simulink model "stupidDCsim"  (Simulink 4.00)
settings: Solver=ode45  SolverMode=SingleTasking  StartTime=0.0  StopTime=100  RelTol=1e-3  AbsTol=1e-6
PostLoadFcn:
  | stupidDCpostloadfcn
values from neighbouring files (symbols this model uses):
  Ts = 0.01    [pidDCpostloadfcn.m]    (also in stupidDCpostloadfcn.m = 0.1)
undefined symbols (not defined in the file or in its folder): conv, polyc2d, polyval
libraries: adaptlib x3, simulink3 x1

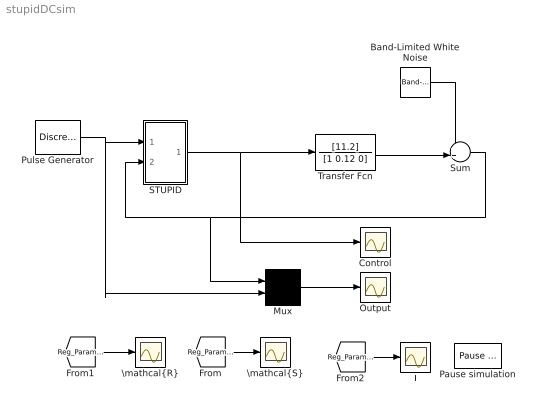
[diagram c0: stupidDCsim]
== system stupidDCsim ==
  Band-Limited White Noise : simulink3/Sources/Band-Limited White Noise  Cov=[0.0001]  Ts=0.1  seed=[23341]
  Control : Scope
  Mux : Mux  Inputs=2
  Output : Scope
  Pause simulation : adaptlib/Pause simulation  par=[50]
  Pulse Generator : DiscretePulseGenerator  PulseType=Time-based  Amplitude=2  Period=10  PulseWidth=50  PhaseDelay=0  SampleTime=1
  STUPID : Subsystem  mask{wo=5, zeta=1, theta0=[0.3;0.1;2; -2], P0=1000*diag([1 1 1 1]), lambda=, a_o=, h=Ts, d0=, um=10}
      mask prompts: wo "w_o (closed loop bandwidth)"; zeta "Closed loop damping"; theta0 "Initial estimate"; P0 "Initial covariance matrix"; lambda "Forgeting factor"; a_o "Observer pole"; h "Sampling time"; d0 "d0 (prediction horizon)"; um "Maximum control signal"
      mask help: DSTR with integral term.
      mask init:
      | Ts=0.1;
  Sum : Sum  Inputs=++|  SaturateOnIntegerOverflow=on
  T : Scope
  Transfer Fcn : TransferFcn  Numerator=[11.2]  Denominator=[1 0.12 0]  AbsoluteTolerance=auto  Realization=auto
  "\\mathcal{R}" : Scope
  "\\mathcal{S}" : Scope
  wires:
  Mux/1 -> Output/1
  Pulse Generator/1 -> Mux/2, STUPID/1(u_c)
  STUPID/1(u) -> Control/1, Transfer Fcn/1
  Transfer Fcn/1 -> Sum/2
  Sum/1 -> STUPID/2(y), Mux/1
  Band-Limited White Noise/1 -> Sum/1
  [Reg_ParametersStilde] -> "\\mathcal{S}"/1
  [Reg_ParametersRtilde] -> "\\mathcal{R}"/1
  [Reg_ParametersT] -> T/1

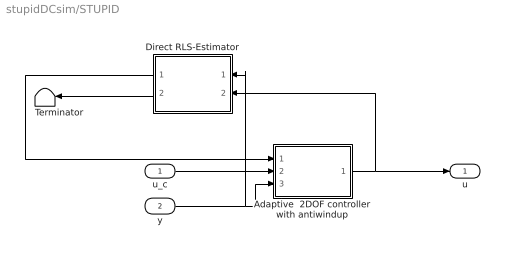
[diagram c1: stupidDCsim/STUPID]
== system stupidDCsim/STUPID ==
  u_c : Inport  Port=1  LatchInput=off
  y : Inport  Port=2  LatchInput=off
  Adaptive  2DOF controller with antiwindup : Subsystem  AncestorBlock=|  mask{n_r=2, ulim=um, A_m=polyc2d([1 2*zeta*wo wo^2],h), A_o=[1 -a_o], A_ow=polyc2d([1 2*0.7*7 7^2],h), h=h}
      | adaptlib/Adaptive 
      | 2DOF controller
      | with antiwindup
      mask prompts: n_r "n_r (degree of R, S and T)"; ulim "Maximum control signal"; A_o "A_o (Observer polynomial)"; A_ow "A_ow (Anti windup polynomial)"; h "Sampling period"
      mask help: A two-degree-of-freedom linear controller with control signal saturation and anti windup. A_o(q)v(k)=T(q)u_c(k)-S(q)y(k)-(A_o(q)-R(q))u(t) u(k)=f(v(k))
  Direct RLS-Estimator : Subsystem  Orientation=left  Priority=1  AncestorBlock=adaptlib/Direct RLS-Estimator  mask{n_r=1, theta_0=theta0, P_0=P0, lambda=lambda, A_m=polyc2d([1 2*zeta*wo wo^2],h), A_o=[1 -a_o], d0=d0, h=h}
      mask prompts: n_r "n_r (degree of estimated R, S )"; theta_0 "Initial estimate"; P_0 "Initial covariance matrix"; h "Sampling period"
  Terminator : Terminator
  u : Outport  Port=1
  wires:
  Direct RLS-Estimator/2(P) -> Terminator/1
  Direct RLS-Estimator/1("[R,S,T]") -> Adaptive  2DOF controller with antiwindup/1("[R,S,T]")
  u_c/1 -> Adaptive  2DOF controller with antiwindup/2(u_c)
  y/1 -> Adaptive  2DOF controller with antiwindup/3(y), Direct RLS-Estimator/1(y)
  Adaptive  2DOF controller with antiwindup/1(u) -> Direct RLS-Estimator/2(u), u/1

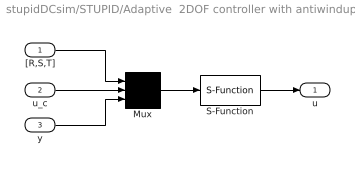
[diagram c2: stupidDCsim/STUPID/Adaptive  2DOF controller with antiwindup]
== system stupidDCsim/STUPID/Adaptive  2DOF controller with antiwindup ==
  "[R,S,T]" : Inport  Port=1  LatchInput=off
  u_c : Inport  Port=2  LatchInput=off
  y : Inport  Port=3  LatchInput=off
  Mux : Mux  Inputs=3
  S-Function : S-Function  FunctionName=rstdirint  Parameters=2,h,A_o,A_ow,A_m,ulim  PortCounts=[]  SFunctionModules=''
  u : Outport  Port=1  InitialOutput=0
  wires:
  "[R,S,T]"/1 -> Mux/1
  y/1 -> Mux/3
  Mux/1 -> S-Function/1
  S-Function/1 -> u/1
  u_c/1 -> Mux/2

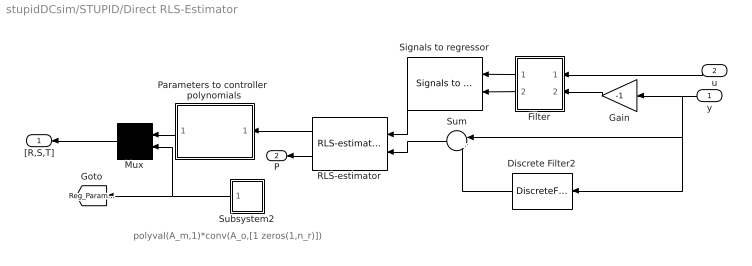
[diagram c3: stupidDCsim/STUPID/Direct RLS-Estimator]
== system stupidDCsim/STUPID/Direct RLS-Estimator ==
  note: polyval(A_m,1)*conv(A_o,[1 zeros(1,n_r)])
  y : Inport  Orientation=left  Port=1  LatchInput=off
  u : Inport  Orientation=left  Port=2  LatchInput=off
  Discrete Filter2 : DiscreteFilter  Orientation=left  Numerator=[zeros(1,d0) 1]*polyval(A_m,1)*polyval(A_o,1)  Denominator=conv(A_m,A_o)  SampleTime=h  Realization=auto
  Filter : Subsystem  Orientation=left  mask{A_m=A_m, A_o=A_o, d0=d0, h=h}
  Gain : Gain  Orientation=left  Gain=-1  Multiplication=Element-wise(K.*u)  SaturateOnIntegerOverflow=on
  Mux : Mux  Orientation=left  Inputs=2
  Parameters to controller  polynomials : Subsystem  Orientation=left  AncestorBlock="adaptlib/Parameters to controller  polynomials"  mask{n_r=n_r}
      mask prompts: n_r "n_r (degree of R, S )"
  RLS-estimator : adaptlib/RLS-estimator  Orientation=left  n=2*(n_r+1)  theta_0=theta_0  P_0=P_0  lambda=lambda  h=h
  Signals to regressor : adaptlib/Signals to regressor  Orientation=left  m=n_r+1  n=n_r+1  h=h
  Subsystem2 : Subsystem  Orientation=left
  Sum : Sum  Orientation=left  Inputs=|+-  SaturateOnIntegerOverflow=on
  "[R,S,T]" : Outport  Orientation=left  Port=1  InitialOutput=0
  P : Outport  Orientation=left  Port=2  InitialOutput=0
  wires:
  Mux/1 -> "[R,S,T]"/1
  Gain/1 -> Filter/2(y)
  u/1 -> Filter/1(u)
  y/1 -> Gain/1, Sum/1, Discrete Filter2/1
  Filter/1(u_f) -> Signals to regressor/1
  Filter/2(y_f) -> Signals to regressor/2
  Signals to regressor/1 -> RLS-estimator/1
  RLS-estimator/2 -> P/1
  RLS-estimator/1 -> Parameters to controller  polynomials/1(theta)
  Parameters to controller  polynomials/1("[R,S]") -> Mux/1
  Sum/1 -> RLS-estimator/2
  Discrete Filter2/1 -> Sum/2
  Subsystem2/1(Out1) -> Mux/2, [Reg_ParametersT]

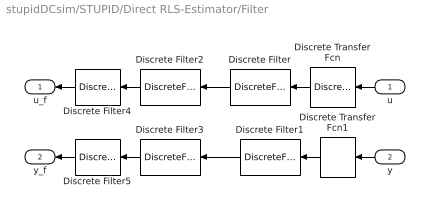
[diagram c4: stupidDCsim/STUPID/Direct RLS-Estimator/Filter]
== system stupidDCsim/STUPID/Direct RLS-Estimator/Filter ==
  u : Inport  Orientation=left  Port=1  LatchInput=off
  y : Inport  Orientation=left  Port=2  LatchInput=off
  Discrete Transfer Fcn : DiscreteTransferFcn  Orientation=left  Numerator=[1]  Denominator=[1 zeros(1,d0) ]  SampleTime=h  Realization=auto
  Discrete Transfer Fcn1 : DiscreteTransferFcn  Orientation=left  Numerator=[1]  Denominator=[1 zeros(1,d0) ]  SampleTime=h  Realization=auto
  Discrete Filter : DiscreteFilter  Orientation=left  Numerator=[1]  Denominator=A_o  SampleTime=h  Realization=auto
  Discrete Filter1 : DiscreteFilter  Orientation=left  Numerator=[1]  Denominator=A_o  SampleTime=h  Realization=auto
  Discrete Filter2 : DiscreteFilter  Orientation=left  Numerator=[1]  Denominator=A_m  SampleTime=h  Realization=auto
  Discrete Filter3 : DiscreteFilter  Orientation=left  Numerator=[1]  Denominator=A_m  SampleTime=h  Realization=auto
  Discrete Filter4 : DiscreteFilter  Orientation=left  Numerator=[1 -1]  Denominator=[1]  SampleTime=h  Realization=auto
  Discrete Filter5 : DiscreteFilter  Orientation=left  Numerator=[1 -1]  Denominator=[1 ]  SampleTime=h  Realization=auto
  u_f : Outport  Orientation=left  Port=1  InitialOutput=0
  y_f : Outport  Orientation=left  Port=2  InitialOutput=0
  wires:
  Discrete Filter2/1 -> Discrete Filter4/1
  Discrete Filter3/1 -> Discrete Filter5/1
  u/1 -> Discrete Transfer Fcn/1
  y/1 -> Discrete Transfer Fcn1/1
  Discrete Filter/1 -> Discrete Filter2/1
  Discrete Filter1/1 -> Discrete Filter3/1
  Discrete Transfer Fcn/1 -> Discrete Filter/1
  Discrete Transfer Fcn1/1 -> Discrete Filter1/1
  Discrete Filter4/1 -> u_f/1
  Discrete Filter5/1 -> y_f/1

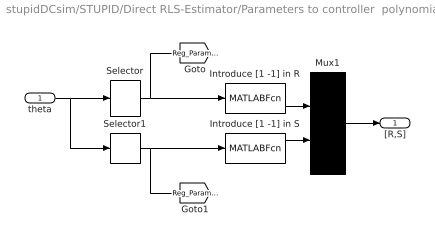
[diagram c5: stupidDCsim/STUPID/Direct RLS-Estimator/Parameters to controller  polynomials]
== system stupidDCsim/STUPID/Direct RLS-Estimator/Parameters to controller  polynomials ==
  theta : Inport  Port=1  LatchInput=off
  Introduce [1 -1] in R : MATLABFcn  MATLABFcn=conv(u,[1 -1])  OutputDimensions=3  OutputSignalType=auto  Output1D=on
  Introduce [1 -1] in S : MATLABFcn  MATLABFcn=conv(u,[1 -1])  OutputDimensions=3  OutputSignalType=auto  Output1D=on
  Mux1 : Mux  Inputs=2
  Selector : Selector  InputType=Vector  ElementSrc=Internal  Elements=[1 : n_r+1]  RowSrc=Internal  Rows=1  ColumnSrc=Internal  Columns=1  InputPortWidth=2*(n_r+1)
  Selector1 : Selector  InputType=Vector  ElementSrc=Internal  Elements="[n_r+2 :  2*(n_r+1)]"  RowSrc=Internal  Rows=1  ColumnSrc=Internal  Columns=1  InputPortWidth=2*(n_r+1)
  "[R,S]" : Outport  Port=1  InitialOutput=0
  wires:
  Selector1/1 -> Introduce [1 -1] in S/1, [Reg_ParametersStilde]
  Mux1/1 -> "[R,S]"/1
  Selector/1 -> Introduce [1 -1] in R/1, [Reg_ParametersRtilde]
  theta/1 -> Selector/1, Selector1/1
  Introduce [1 -1] in R/1 -> Mux1/1
  Introduce [1 -1] in S/1 -> Mux1/2

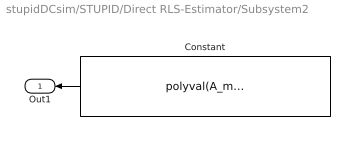
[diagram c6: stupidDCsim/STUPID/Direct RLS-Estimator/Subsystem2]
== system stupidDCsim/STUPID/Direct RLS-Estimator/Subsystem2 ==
  Constant : Constant  Orientation=left  Value=polyval(A_m,1)*conv(A_o,[1 zeros(1,n_r)])
  Out1 : Outport  Orientation=left  Port=1
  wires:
  Constant/1 -> Out1/1
